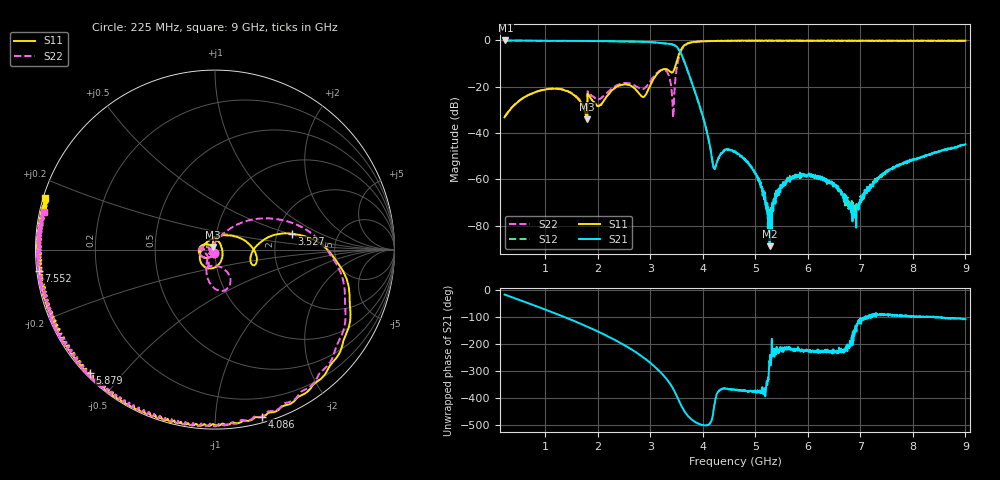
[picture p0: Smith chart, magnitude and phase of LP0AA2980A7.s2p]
!Agilent Technologies,E8358A,US41080443,A.07.50.56
!Agilent E8358A: A.07.50.56
!Date: Tuesday, January 09, 2018 21:47:00
!Correction: S11(Full 2 Port(1,2))
!S21(Full 2 Port(1,2))
!S12(Full 2 Port(1,2))
!S22(Full 2 Port(1,2))
!S2P File: Measurements: S11, S21, S12, S22:
# Hz S  dB  R 50
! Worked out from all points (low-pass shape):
!   1601 points, 225 MHz to 9 GHz, reference 50 ohm
!   highest |S21| = -0.02 dB at 241.5 MHz (marker M1); lowest = -88.8 dB at 5.271 GHz (marker M2)
!   |S21| within 3 dB of the highest: start of sweep to 3.514 GHz
!   lowest |S11| = -34.0 dB at 1.799 GHz (marker M3), VSWR 1.04, Z = 48.6 + j1.41 ohm
!   |S11| at or under -10 dB: start of sweep to 3.491 GHz
!   |S22| runs from -33.3 to 0.0 dB; largest |S21 - S12| = 0.0082
!   S11 on the Smith chart (normalised r, x): 225 MHz: 0.99, -0.04; 3.527 GHz: 2.41, +0.53; 4.086 GHz: 0.04, -1.32; 5.879 GHz: 0.01, -0.41; 7.552 GHz: 0.01, -0.06; 9 GHz: 0.01, +0.15
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2.25e8  -33.16 -101.9  -0.03 -16.2  -0.08 -16.2  -33.01 -105.7
2.414531e8  -32.54 -102.8  -0.02 -17.4  -0.08 -17.4  -32.42 -107.5
1.01475e9  -21.10 -160.8  -0.16 -73.2  -0.22 -73.1  -21.05 -161.7
1.689328e9  -27.15 141.1  -0.22 -126.0  -0.28 -125.9  -26.54 163.1
1.799016e9  -34.05 132.9  -0.23 -135.4  -0.28 -135.3  -32.18 174.5
2.511984e9  -18.97 -117.7  -0.44 155.0  -0.49 155.2  -18.35 -114.5
2.873953e9  -24.37 118.5  -0.59 109.1  -0.64 109.4  -20.89 -84.5
3.153656e9  -13.87 5.0  -1.01 63.0  -1.06 63.1  -13.48 -66.8
3.427875e9  -13.73 -5.1  -1.74 -3.8  -1.79 -3.7  -30.21 -157.5
3.526594e9  -7.21 11.7  -3.41 -43.1  -3.44 -42.8  -9.06 29.5
3.680156e9  -1.64 -24.4  -11.15 -98.1  -11.22 -98.0  -1.84 -26.1
4.086e9  -0.28 -74.4  -40.12 -141.3  -40.25 -140.5  -0.25 -78.7
4.223109e9  -0.22 -83.1  -55.52 -61.9  -55.12 -64.7  -0.17 -87.0
4.6125e9  -0.11 -100.5  -47.88 -10.6  -48.05 -9.8  -0.08 -103.1
5.040281e9  -0.15 -113.7  -58.60 -17.7  -59.49 -14.8  -0.20 -115.8
5.270625e9  -0.10 -120.7  -88.78 99.1  -73.02 36.9  -0.04 -121.8
5.879391e9  -0.20 -135.4  -57.92 135.0  -58.19 136.0  -0.12 -137.2
6.076828e9  -0.21 -140.5  -58.75 130.7  -58.64 133.1  -0.10 -141.9
6.883031e9  -0.16 -158.8  -74.63 -168.7  -75.29 -142.7  -0.22 -159.5
7.541156e9  -0.15 -172.7  -56.06 -93.9  -56.26 -90.5  -0.23 -171.6
7.552125e9  -0.09 -173.2  -55.76 -92.2  -56.01 -92.3  -0.22 -171.3
9e9  -0.10 163.2  -44.79 -107.8  -44.97 -106.9  -0.21 167.5
